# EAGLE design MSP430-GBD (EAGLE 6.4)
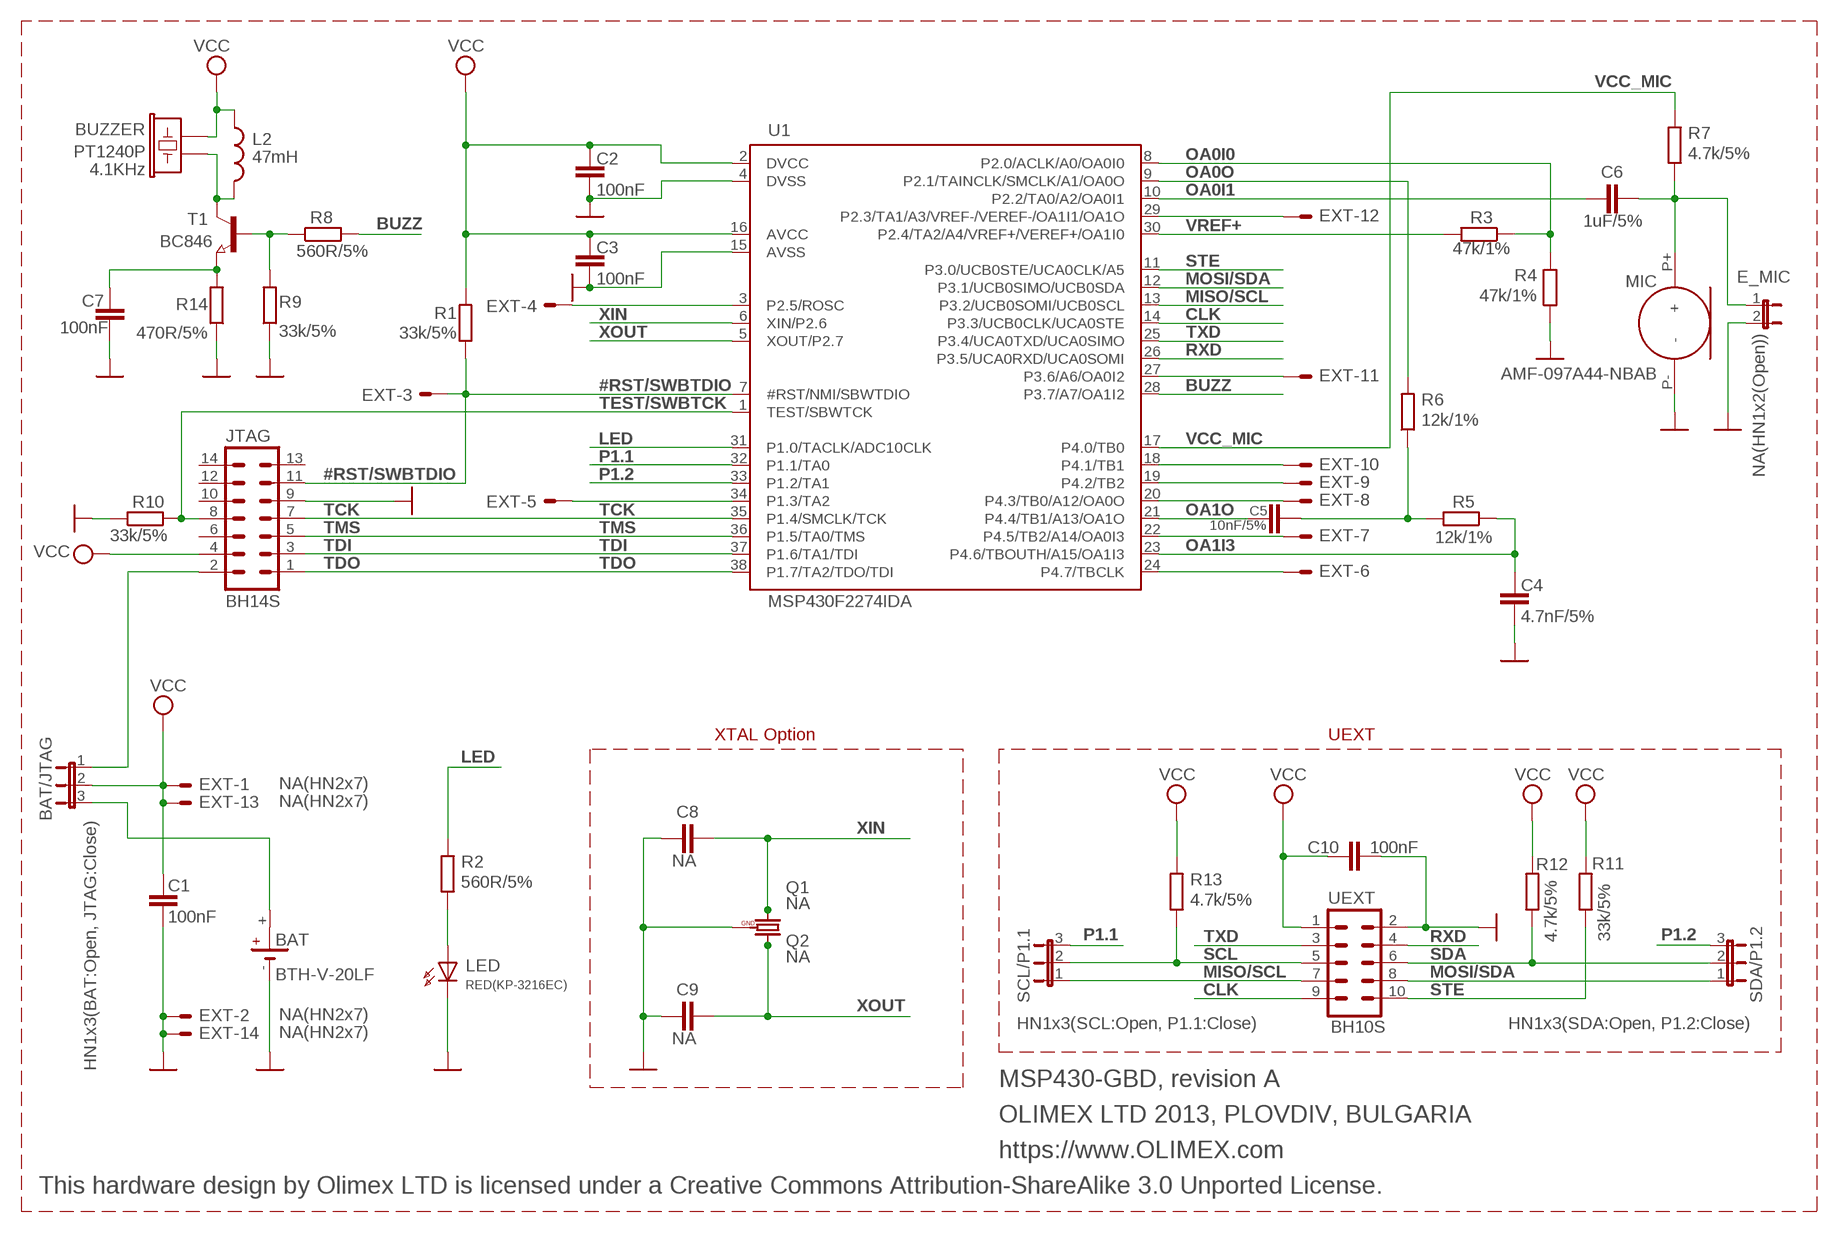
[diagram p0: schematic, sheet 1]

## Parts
BAT  BTH-V-20LF  B1  [3V_BAT_HOLDER]
BAT/JTAG  HN1x3(BAT:Open, JTAG:Close)  JP2E  [JP2]
BUZZER  PT1240P  BUZ3  [BUZ14MM]
C1  100nF  C-EUC0603  [C0603]
C2  100nF  C-EUC0603  [C0603]
C3  100nF  C-EUC0603  [C0603]
C4  4.7nF/5%  C-EUC0603  [C0603]
C5  10nF/5%  C-EUC0603  [C0603]
C6  1uF/5%  C-EUC0603  [C0603]
C7  100nF  C-EUC0603  [C0603]
C8  NA  C-EUC0603  [C0603]
C9  NA  C-EUC0603  [C0603]
C10  100nF  C-EUC0603  [C0603]
E_MIC  NA(HN1x2(Open))  JP1E  [JP1]
EXT  NA(HN2x7)  ML14ML14_NO_FRAMEE  [ML14_NO_FRAME]
JTAG  BH14S  ML14  [ML14]
L2  47mH  LSW68  [SW68]
LED  RED(KP-3216EC)  LED2  [SMD_LED]
MIC  AMF-097A44-NBAB  MICR  [MIC]
Q1  NA  HC49/S2  [HC49/SMD2]
Q2  NA  Q_GNDTC38H_SMD_GND  [TC38H_SMD_GND]
R1  33k/5%  R-EU_R0603  [R0603]
R2  560R/5%  R-EU_R0603  [R0603]
R3  47k/1%  R-EU_R0603  [R0603]
R4  47k/1%  R-EU_R0603  [R0603]
R5  12k/1%  R-EU_R0603  [R0603]
R6  12k/1%  R-EU_R0603  [R0603]
R7  4.7k/5%  R-EU_R0603  [R0603]
R8  560R/5%  R-EU_R0603  [R0603]
R9  33k/5%  R-EU_R0603  [R0603]
R10  33k/5%  R-EU_R0603  [R0603]
R11  33k/5%  R-EU_R0603  [R0603]
R12  4.7k/5%  R-EU_R0603  [R0603]
R13  4.7k/5%  R-EU_R0603  [R0603]
R14  470R/5%  R-EU_R1206_5MIL_WS  [R1206_5MIL_WS]
SCL/P1.1  HN1x3(SCL:Open, P1.1:Close)  JP2E  [JP2]
SDA/P1.2  HN1x3(SDA:Open, P1.2:Close)  JP2E  [JP2]
T1  BC846  NPN-TRANSISTOR_SOT23  [SOT23]
U1  MSP430F2274IDA  MSP430F2274  [TSSOP38]
UEXT  BH10S  ML10  [ML10]

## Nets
#RST/SWBTDIO: EXT.3 JTAG.11 R1.1 U1.7(#RST/NMI/SBWTDIO)
BUZZ: R8.2 U1.28(P3.7/A7/OA1I2)
CLK: U1.14(P3.3/UCB0CLK/UCA0STE) UEXT.9
GND: BAT.- C1.2 C2.2 C3.2 C4.2 C7.1 C8.1 C9.1 C10.2 E_MIC.2 EXT.2 EXT.14 JTAG.9 LED.C MIC.P-(-) Q2.GND R4.1 R9.1 R10.1 R14.1 U1.4(DVSS) U1.15(AVSS) UEXT.2
LED: R2.2 U1.31(P1.0/TACLK/ADC10CLK)
MISO/SCL: SCL/P1.1.1 U1.13(P3.2/UCB0SOMI/UCB0SCL) UEXT.7
MOSI/SDA: SDA/P1.2.1 U1.12(P3.1/UCB0SIMO/UCB0SDA) UEXT.8
N$1: BAT.+ BAT/JTAG.3
N$2: BAT/JTAG.1 JTAG.2
N$3: EXT.4 U1.3(P2.5/ROSC)
N$4: LED.A R2.1
N$6: C6.2 E_MIC.1 MIC.P+(+) R7.1
N$7: C5.2 R5.2 R6.1
N$9: R8.1 R9.2 T1.1(B)
N$10: C7.2 R14.2 T1.2(E)
N$14: EXT.5 U1.34(P1.3/TA2)
N$19: EXT.6 U1.24(P4.7/TBCLK)
N$20: BUZZER.+ L2.2 T1.3(C)
N$21: EXT.7 U1.22(P4.5/TB2/A14/OA0I3)
N$22: EXT.8 U1.20(P4.3/TB0/A12/OA0O)
N$23: EXT.9 U1.19(P4.2/TB2)
N$24: EXT.10 U1.18(P4.1/TB1)
N$25: EXT.11 U1.27(P3.6/A6/OA0I2)
N$26: EXT.12 U1.29(P2.3/TA1/A3/VREF-/VEREF-/OA1I1/OA1O)
OA0I0: R3.1 R4.2 U1.8(P2.0/ACLK/A0/OA0I0)
OA0I1: C6.1 U1.10(P2.2/TA0/A2/OA0I1)
OA0O: R6.2 U1.9(P2.1/TAINCLK/SMCLK/A1/OA0O)
OA1I3: C4.1 R5.1 U1.23(P4.6/TBOUTH/A15/OA1I3)
OA1O: C5.1 U1.21(P4.4/TB1/A13/OA1O)
P1.1: SCL/P1.1.3 U1.32(P1.1/TA0)
P1.2: SDA/P1.2.3 U1.33(P1.2/TA1)
RXD: U1.26(P3.5/UCA0RXD/UCA0SOMI) UEXT.4
SCL: R13.1 SCL/P1.1.2 UEXT.5
SDA: R12.1 SDA/P1.2.2 UEXT.6
STE: R11.1 U1.11(P3.0/UCB0STE/UCA0CLK/A5) UEXT.10
TCK: JTAG.7 U1.35(P1.4/SMCLK/TCK)
TDI: JTAG.3 U1.37(P1.6/TA1/TDI)
TDO: JTAG.1 U1.38(P1.7/TA2/TDO/TDI)
TEST/SWBTCK: JTAG.8 R10.2 U1.1(TEST/SBWTCK)
TMS: JTAG.5 U1.36(P1.5/TA0/TMS)
TXD: U1.25(P3.4/UCA0TXD/UCA0SIMO) UEXT.3
VCC: BAT/JTAG.2 BUZZER.- C1.1 C2.1 C3.1 C10.1 EXT.1 EXT.13 JTAG.4 L2.1 R1.2 R11.2 R12.2 R13.2 U1.2(DVCC) U1.16(AVCC) UEXT.1
VCC_MIC: R7.2 U1.17(P4.0/TB0)
VREF+: R3.2 U1.30(P2.4/TA2/A4/VREF+/VEREF+/OA1I0)
XIN: C8.2 Q1.2 Q2.1 U1.6(XIN/P2.6)
XOUT: C9.2 Q1.1 Q2.2 U1.5(XOUT/P2.7)
Unconnected: BAT.1+(+) JTAG.6 JTAG.10 JTAG.12 JTAG.13 JTAG.14

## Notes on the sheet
- PT1240P
- 4.1KHz
- XTAL Option | UEXT
- MSP430-GBD, revision A
- OLIMEX LTD 2013, PLOVDIV, BULGARIA
- https://www.OLIMEX.com
- This hardware design by Olimex LTD is licensed under a Creative Commons Attribution-ShareAlike 3.0 Unported License.

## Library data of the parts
BAT = DOUBLE-SIDE:B: LI BATTERY Varta
BAT/JTAG SCL/P1.1 SDA/P1.2 = jumper:JP2E: JUMPER
BUZZER = gogo:BUZ
C1-C10 = rcl:C-EU: CAPACITOR, European symbol
E_MIC = jumper:JP1E: JUMPER
EXT = con-harting-ml:ML14?E: HARTING
JTAG = con-harting-ml:ML14: HARTING
L2 = DOUBLE-SIDE:L
LED = DOUBLE-SIDE:LED
MIC = DOUBLE-SIDE:MIC: ELECTRETE MICROPHONE
Q1 = crystal:HC49/S: CRYSTAL
Q2 = crystal:Q_GND
R1-R14 = rcl:R-EU_: RESISTOR, European symbol
T1 = semicon-smd-ipc:NPN-TRANSISTOR_: NPN TRANSISTOR
U1 = OLIMEX_IC:MSP430F2274
UEXT = con-harting-ml:ML10: HARTING

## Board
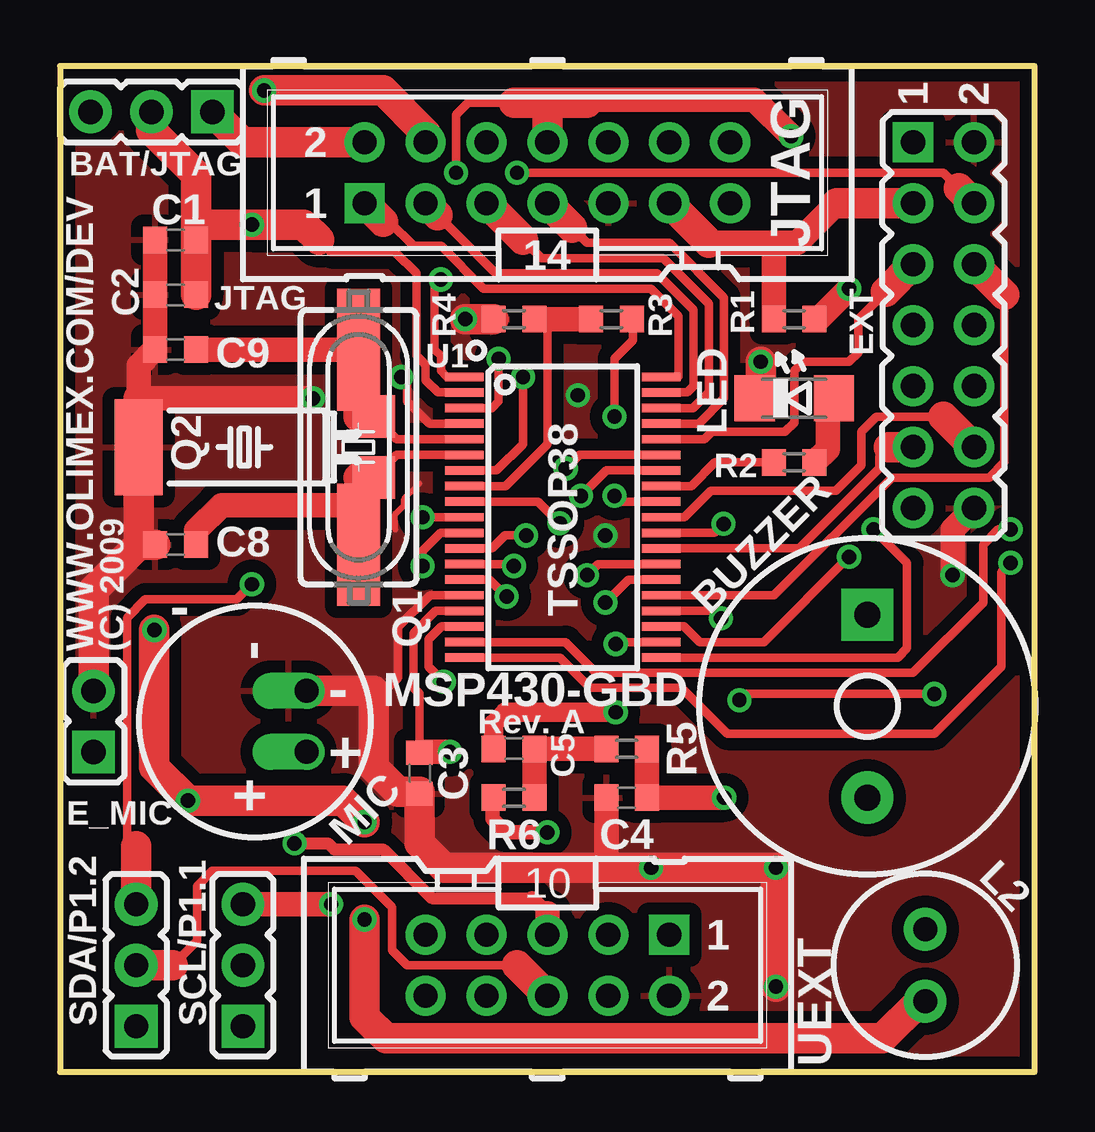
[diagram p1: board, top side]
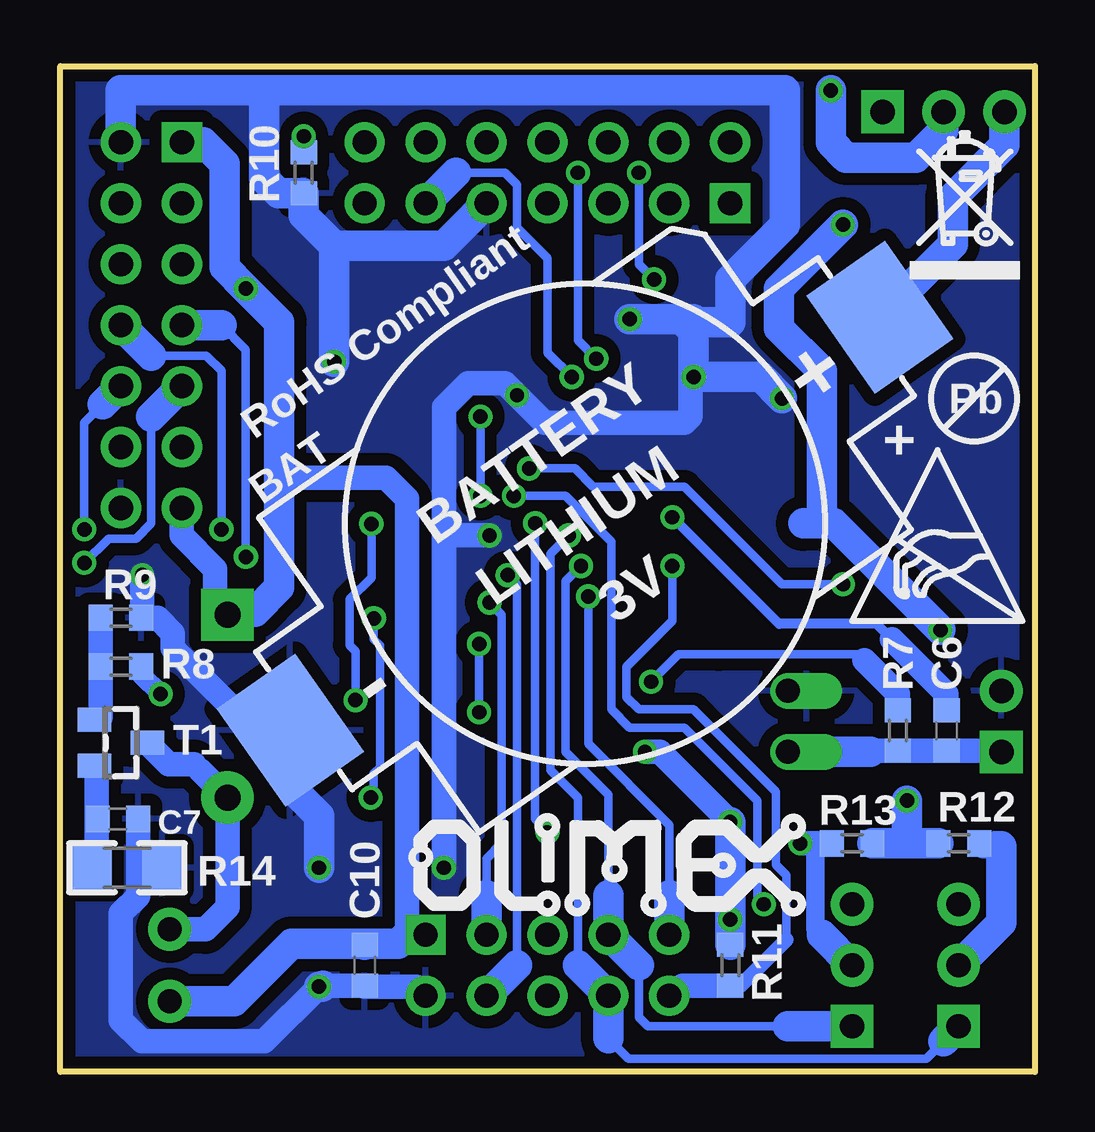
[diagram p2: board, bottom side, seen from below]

Size 40.62 x 41.91 mm. Coordinates in mm from the lower left corner, seen from the top.
Outline: 0.01,0 40.62,0 40.62,41.91 0.01,41.91 0,41.91 0,0.01 0.01,0
Copper layers (1+16): Top 0.035mm / dielectric 1.5mm / Bottom 0.035mm
Design rules "default": minimum track width 10mil, minimum drill 23mil, track to track 10mil, track to pad 10mil, pad to pad 10mil, via to via 10mil, smd to smd 0mil, copper to edge 10mil, drill to drill 10mil, minimum pad ring 10mil, minimum via ring 8mil, stop-mask expansion 4mil, vias tented up to drill 25mil, thermal gap 20mil

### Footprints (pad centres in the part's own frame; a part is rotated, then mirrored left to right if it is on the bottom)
3V_BAT_HOLDER = smd 2 x 2: 1+ -15,0 | smd 4 x 5: + -15,0; - 15,0
JP2 = drill 1.016 pad 1.778 square: 1 -2.54,0 | drill 1.016 pad 1.778: 2 0,0; 3 2.54,0
BUZ14MM = drill 1.092 pad 2.184: + 3.81,0 | drill 1.092 pad 2.184 square: - -3.81,0
C0603 = smd 1 x 1.1: 1 -0.85,0; 2 0.85,0
JP1 = drill 1.016 pad 1.778 square: 1 0,-1.27 | drill 1.016 pad 1.778: 2 0,1.27
ML14_NO_FRAME = drill 1.016 pad 1.676 square: 1 -7.62,-1.27 | drill 1.016 pad 1.676: 2 -7.62,1.27; 3 -5.08,-1.27; 4 -5.08,1.27; 5 -2.54,-1.27; 6 -2.54,1.27; 7 0,-1.27; 8 0,1.27; 9 2.54,-1.27; 10 2.54,1.27; 11 5.08,-1.27; 12 5.08,1.27; 13 7.62,-1.27; 14 7.62,1.27
ML14 = drill 1.016 pad 1.676 square: 1 -7.62,-1.27 | drill 1.016 pad 1.676: 2 -7.62,1.27; 3 -5.08,-1.27; 4 -5.08,1.27; 5 -2.54,-1.27; 6 -2.54,1.27; 7 0,-1.27; 8 0,1.27; 9 2.54,-1.27; 10 2.54,1.27; 11 5.08,-1.27; 12 5.08,1.27; 13 7.62,-1.27; 14 7.62,1.27
SW68 = drill 1 pad 1.778: 1 -1.5,0; 2 1.5,0
SMD_LED = smd 1.676 x 1.93: A 1.65,0; C -1.65,0
MIC = drill 1 offset: P+ -1.27,-2.159; P- 1.27,-2.159
HC49/SMD2 = smd 5.08 x 1.778: 1 -4.064,0; 2 4.064,0
TC38H_SMD_GND = smd 1.778 x 1.778: 1 -1.27,-3.81; 2 1.27,-3.81 | smd 4 x 2: GND 0,6
R0603 = smd 1 x 1.1: 1 -0.85,0; 2 0.85,0
R1206_5MIL_WS = smd 1.651 x 1.778: 1 -1.46,0; 2 1.46,0
SOT23 = smd 1 x 1.4: 1 -0.95,-1.1; 2 0.95,-1.1; 3 0,1.1
TSSOP38 = smd 0.35 x 1.6: 1 -5.85,-4.1; 2 -5.2,-4.1; 3 -4.55,-4.1; 4 -3.9,-4.1; 5 -3.25,-4.1; 6 -2.6,-4.1; 7 -1.95,-4.1; 8 -1.3,-4.1; 9 -0.65,-4.1; 10 0,-4.1; 11 0.65,-4.1; 12 1.3,-4.1; 13 1.95,-4.1; 14 2.6,-4.1; 15 3.25,-4.1; 16 3.9,-4.1; 17 4.55,-4.1; 18 5.2,-4.1; 19 5.85,-4.1; 20 5.85,4.1; 21 5.2,4.1; 22 4.55,4.1; 23 3.9,4.1; 24 3.25,4.1; 25 2.6,4.1; 26 1.95,4.1; 27 1.3,4.1; 28 0.65,4.1; 29 0,4.1; 30 -0.65,4.1; 31 -1.3,4.1; 32 -1.95,4.1; 33 -2.6,4.1; 34 -3.25,4.1; 35 -3.9,4.1; 36 -4.55,4.1; 37 -5.2,4.1; 38 -5.85,4.1
ML10 = drill 1.016 pad 1.676 square: 1 -5.08,-1.27 | drill 1.016 pad 1.676: 2 -5.08,1.27; 3 -2.54,-1.27; 4 -2.54,1.27; 5 0,-1.27; 6 0,1.27; 7 2.54,-1.27; 8 2.54,1.27; 9 5.08,-1.27; 10 5.08,1.27

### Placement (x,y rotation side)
BAT  18.75,22.84 215 bottom
BAT/JTAG  3.81,40.01 180 top
BUZZER  33.66,15.24 270 top
C1  4.83,34.67 180 top
C2  4.83,32.38 180 top
C3  14.99,12.45 270 top
C4  23.62,11.43 180 top
C5  18.92,13.46 0 top
C6  3.68,14.22 270 bottom
C7  38.23,10.54 180 bottom
C8  4.83,21.97 0 top
C9  4.83,30.1 0 top
C10  27.94,4.45 270 bottom
E_MIC  1.4,14.61 0 top
EXT  36.83,31.11 270 top
JTAG  20.32,37.47 0 top
L2  36.07,4.45 90 top
LED  30.61,28.07 0 top
MIC  8.13,14.61 90 top
Q1  12.45,26.04 270 top
Q2  9.27,26.04 90 top
R1  30.61,31.37 0 top
R2  30.61,25.4 180 top
R3  22.99,31.37 0 top
R4  18.92,31.37 0 top
R5  23.62,13.46 180 top
R6  18.92,11.43 180 top
R7  5.71,14.22 90 bottom
R8  38.1,16.89 0 bottom
R9  38.1,18.92 180 bottom
R10  30.48,37.47 90 bottom
R11  12.7,4.45 90 bottom
R12  3.17,9.53 180 bottom
R13  7.62,9.53 0 bottom
R14  37.85,8.51 180 bottom
SCL/P1.1  7.62,4.45 90 top
SDA/P1.2  3.17,4.45 90 top
T1  38.1,13.72 270 bottom
U1  20.95,23.11 270 top
U$1  [RECYCLE_BIN1/8]  5.21,33.02 0 bottom
U$3  [PB_SMALL]  2.54,28.07 0 bottom
U$4  [ESD_SYMBOL]  7.62,18.8 0 bottom
U$6  [OLIMEX_LOGO1_V]  8.38,6.35 0 bottom
UEXT  20.32,4.45 180 top

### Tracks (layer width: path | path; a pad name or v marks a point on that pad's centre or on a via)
#RST/SWBTDIO  (via drill 0.6)
  Top 0.356: U1.7 18.21,25.06 19.3,26.16 v19.3,28.96
  Top 1.016: 27.05,34.54 29.76,34.54 | 29.76,34.54 30.73,34.54 32.38,36.2 | 29.76,34.54 R1.1
  Top 1.27: JTAG.11 27.05,34.54 | 32.38,36.2 EXT.3
  Bottom 0.356: 24.13,37.47 22.1,37.47 21.59,36.96 21.59,35.18 20.32,33.91 20.32,29.97 v19.3,28.96
  Bottom 1.27: 24.13,37.47 JTAG.11
BUZZ  (via drill 0.6)
  Top 0.356: U1.28 27.29,22.46 v27.66,22.84 | v28.32,15.49 28.57,15.75 v36.45,15.75
  Bottom 0.356: v28.32,15.49 28.32,17.53 28.57,17.78 28.57,19.68 27.66,20.6 v27.66,22.84
  Bottom 0.813: v36.45,15.75 37.25,16.55 R8.2
CLK  (via drill 0.6)
  Top 0.356: U1.14 17.92,20.51 v18.62,19.81
  Bottom 0.356: v18.62,19.81 18.62,13.66 15.24,10.29 15.24,7.37
  Bottom 1.27: UEXT.9 15.24,7.37
GND  (via drill 0.6)
  Top 0.254: 14.99,24.51 14.35,23.88 14.35,23.62 13.97,23.24 13.97,22.61
  Top 0.356: U1.4 15.4,27.01 14.48,27.94 14.48,28.7 v14.22,28.96 | U1.15 15.42,19.86 14.1,18.54 14.1,16.43 13.54,15.88 13.08,15.88
  Top 1.016: C1.2 C2.2 C9.1 3.94,30.1 3.27,29.43 3.27,28.07 v10.54,28.07 | 29.21,28.07 LED.C | 22.73,8.51 22.77,8.51 C4.2 | EXT.14 37.21,22.61 v37.21,20.7
  Top 1.27: 3.27,28.07 Q2.GND 3.27,21.97 | 3.27,21.97 C8.1 | 3.27,21.97 1.4,20.1 E_MIC.2 | v29.21,29.59 29.21,28.07 | v29.84,3.56 v29.84,8.51 v24.64,8.51 22.73,8.51 16,8.51 14.99,9.53 C3.2 14.99,11.68 14.1,11.68 13.08,12.7 13.08,15.88 MIC.P- | v16.89,31.37 R4.1
  Bottom 0.356: 38.1,2.16 38.1,2.29
  Bottom 0.813: 28.16,3.6 28.07,3.68 27.98,3.6 C10.2 27.94,3.56 | 23.5,28.7 23.62,28.7
  Bottom 1.016: 37.21,18.92 36.58,18.92 35.94,18.29 35.94,17.65 32.53,14.24 BAT.- | v14.22,28.96 14.35,28.96 14.35,27.3 14.61,27.05 20.45,27.05 v21.59,28.19 22.1,28.7 23.5,28.7 | 24.64,22.35 v22.73,22.35 | 24.64,22.35 v24.64,8.51 | v29.84,3.56 32.13,1.27 37.21,1.27 38.1,2.16 | 38.1,2.29 38.1,6.6 37.38,7.33 37.38,8.51 | 37.38,8.51 C7.1 | 37.21,18.92 R9.1 | 37.21,18.92 v37.21,20.7 | 29.68,3.6 28.16,3.6 | UEXT.2 25.78,3.56 27.94,3.56 | 37.38,8.51 R14.1 | 24.64,22.35 24.64,27.69 23.62,28.7
  Bottom 1.27: v10.54,28.07 11.43,28.96 v14.22,28.96 14.22,31.37 14.48,31.37 | 32.13,40.89 10.41,40.89 10.41,35.31 12.7,33.02 12.7,31.24 14.35,31.24 14.48,31.11 14.48,31.37 | 32.13,40.89 38.1,40.89 EXT.2 | 32.13,40.89 32.13,37.21 31.54,36.62 R10.1 30.48,35.69 29.21,34.42 | JTAG.9 24.64,34.42 29.21,34.42 | 14.48,31.37 v16.89,31.37 | 29.21,34.42 v29.21,29.59 | v29.84,8.51 29.84,10.67 30.99,11.81 30.99,14.22 31.02,14.22 BAT.- | v29.84,3.56 29.72,3.56 29.68,3.6
  pour Top (isolate 0.508, rank 3): -2.54,43.18 42.93,43.18 42.93,-2.54 -2.54,-2.54
  pour Bottom (isolate 0.508, rank 3): -2.54,45.72 43.81,45.72 43.81,-2.54 -2.54,-2.54
LED
  Top 0.356: U1.31 26.32,24.41 27.3,25.4 R2.2
MISO/SCL  (via drill 0.6)
  Top 0.356: U1.13 18.85,21.16 18.93,21.08 v18.92,21.08
  Bottom 0.356: v18.92,21.08 19.56,20.45 19.56,13.34 17.78,11.56 17.78,7.37 | 16.51,4.45 16.51,2.29 16.13,1.91 10.29,1.91
  Bottom 1.27: 17.78,7.37 UEXT.7 16.51,4.45 | SCL/P1.1.1 10.29,1.91
MOSI/SDA  (via drill 0.6)
  Top 0.356: U1.12 18,21.81 18.54,22.35 v19.43,22.35
  Bottom 0.356: v19.43,22.35 20.19,21.59 20.19,12.57 19.05,11.43 19.05,4.45 | 3.81,1.27 4.52,0.56 16.94,0.56 17.78,1.4
  Bottom 1.27: 19.05,4.45 UEXT.8 17.78,1.4 | SDA/P1.2.1 3.81,1.27
N$1
  Bottom 1.27: BAT/JTAG.3 1.27,38.61 3.43,36.45 3.43,34.48 BAT.+
N$2
  Top 1.27: BAT/JTAG.1 7.62,38.73 JTAG.2
N$3  (via drill 0.6)
  Top 0.356: U1.3 18.01,27.66 18.29,27.94 v18.29,29.72 | v19.05,37.47 36.83,37.47 37.47,36.83
  Top 1.27: 37.47,36.83 EXT.4
  Bottom 0.356: v18.29,29.72 19.05,30.48 v19.05,37.47
N$4
  Top 1.016: R2.1 32,25.95 32,27.81 LED.A
N$6
  Bottom 1.016: 6.86,13.34 6.82,13.37 R7.1 C6.2 1.82,13.37 1.78,13.34 E_MIC.1
  Bottom 1.27: 6.86,13.34 MIC.P+
N$7
  Top 1.016: R5.2 C5.2 R6.1
N$9
  Bottom 1.016: R9.2 R8.1 38.95,14.77 39.05,14.67 T1.1
N$10
  Bottom 1.016: T1.2 39.12,12.77 39.12,10.29 | R14.2 39.31,8.95 39.12,9.14 39.12,10.29 | 39.12,10.29 39.12,10.54 C7.2 39.08,10.33 39.12,10.29
N$14
  Top 0.356: U1.34 26.87,26.36 27.18,26.67 30.23,26.67 30.61,27.05 30.61,29.21 30.99,29.59 32.89,29.59 33.27,29.97 33.27,31.37 34.42,32.51
  Top 1.27: 34.42,32.51 EXT.5
N$19
  Top 0.356: 39.37,32.38 39.37,25.4 38.73,24.77 34.67,24.77 29.77,19.86 U1.24
  Top 1.27: 39.37,32.38 EXT.6
N$20
  Bottom 0.762: 34.8,12.57 35.05,12.83
  Bottom 1.016: 34.8,12.57 BUZZER.+ 33.66,6.86 34.57,5.95 L2.2 | 35.05,12.83 36.11,12.83 T1.3
N$21  (via drill 0.6)
  Top 0.356: U1.22 26.01,18.56 26.67,17.91 29.34,17.91 v32.89,21.46
  Bottom 0.356: v32.89,21.46 32.89,30.1 33.91,31.11
  Bottom 1.27: 33.91,31.11 EXT.7
N$22  (via drill 0.6)
  Top 0.356: U1.20 34.92,17.26 35.31,17.65 35.31,21.21 v33.91,22.61
  Bottom 0.356: v33.91,22.61 33.91,29.21 34.54,29.84 36.83,29.84
  Bottom 1.27: 36.83,29.84 EXT.8
N$23  (via drill 0.6)
  Top 0.356: U1.19 20.84,17.26 22.1,16 25.91,16 27.81,14.1 36.45,14.1 39.24,16.89 39.24,20.83 v39.62,21.21
  Bottom 0.356: v39.62,21.21 38.61,22.23 37.47,22.23 36.83,22.86 36.83,27.3
  Bottom 1.27: 36.83,27.3 EXT.9
N$24  (via drill 0.6)
  Top 0.356: U1.18 21.07,17.91 22.35,16.64 35.56,16.64 38.48,19.56 38.48,21.97 39.12,22.61 v39.62,22.61
  Bottom 0.356: v39.62,22.61 39.62,27.05 38.86,27.81
  Bottom 1.27: 38.86,27.81 EXT.10
N$25
  Top 0.356: U1.27 30.83,21.81 34.16,25.15 34.16,25.65 34.54,26.04
  Top 1.27: 34.54,26.04 EXT.11
N$26
  Top 0.356: U1.29 26.04,23.11 27.13,24.21 32.33,24.21 33.4,25.27 33.4,26.67 34.04,27.3 36.83,27.3
  Top 1.27: 36.83,27.3 EXT.12
OA0I0
  Top 0.356: U1.8 18.57,24.41 20.32,26.16 20.32,31.37 R4.2
  Top 1.016: R4.2 R3.1
OA0I1  (via drill 0.6)
  Top 0.356: v15.11,23.11 U1.10
  Bottom 0.406: 5.97,18.03 6.6,18.67 10.67,18.67 v15.11,23.11
  Bottom 1.016: C6.1 3.68,15.75 5.97,18.03
OA0O  (via drill 0.6)
  Top 0.356: U1.9 19.92,23.76 v20.83,22.86
  Top 0.61: R6.2 18.07,11.34 18.03,11.3 18.03,10.54 18.59,9.98 v20.32,9.98
  Bottom 0.356: v20.83,22.86 20.83,10.54 20.32,10.03 v20.32,9.98
OA1I3  (via drill 0.6)
  Top 0.356: U1.23 27.24,19.21 v27.56,18.9
  Top 1.016: v27.69,11.43 C4.1 24.47,12.45 R5.1
  Bottom 0.356: v27.56,18.9 27.56,18.03 27.3,17.78 27.3,12.7 27.56,12.45 27.56,11.43 v27.69,11.43
OA1O  (via drill 0.6)
  Top 0.356: U1.21 23.25,17.91 v23.16,17.83
  Top 0.61: v23.16,14.99 23.16,15.06 23.11,15.11 22.99,14.99
  Top 0.813: C5.1 18.07,14.52 18.54,14.99 22.99,14.99
  Bottom 0.356: v23.16,14.99 v23.16,17.83
P1.1  (via drill 0.6)
  Top 0.356: U1.32 22.78,25.06 v21.72,24
  Top 1.016: SCL/P1.1.3 v11.3,6.99
  Bottom 0.356: v11.3,6.99 11.56,7.24 11.56,11.3 14.61,14.35 16.89,14.35 17.65,15.11 17.65,22.1 19.56,24 v21.72,24
P1.2  (via drill 0.6)
  Top 0.356: U1.33 21.65,25.71 v21.08,25.15 | v8,20.32 7.37,19.68 3.56,19.68 2.79,18.92 2.79,9.78 3.17,9.4
  Top 1.27: SDA/P1.2.3 3.17,9.4
  Bottom 0.356: v8,20.32 10.54,20.32 14.61,24.38 18.41,24.38 19.18,25.15 v21.08,25.15
RXD  (via drill 0.6)
  Top 0.356: U1.26 22.43,21.16 v21.97,20.7
  Bottom 0.356: 21.59,4.45 21.59,20.32 v21.97,20.7
  Bottom 1.27: 21.59,4.45 UEXT.4
SCL  (via drill 0.6)
  Top 0.508: 19.68,7.24 15.49,7.24 13.46,9.27 11.43,9.27 11.18,9.53 v9.78,9.53
  Top 0.61: 19.68,7.24 20.32,6.6
  Top 1.016: 20.32,6.6 UEXT.5
  Bottom 0.762: 8.89,5.71 9.14,5.97 9.14,9.53
  Bottom 1.016: v9.78,9.53 9.14,9.53 R13.1
  Bottom 1.27: SCL/P1.1.2 8.89,5.71
SDA
  Top 0.356: 19.05,4.45 14.48,4.45 13.84,5.08 13.84,6.86 12.32,8.38 6.35,8.38 5.71,7.75 5.71,5.46 4.7,4.45
  Top 1.27: 19.05,4.45 UEXT.6 | SDA/P1.2.2 4.7,4.45
  Bottom 1.016: R12.1 2.29,9.53 2.16,9.4 1.65,9.4
  Bottom 1.27: SDA/P1.2.2 1.4,6.22 1.4,9.4 1.65,9.4
STE  (via drill 0.6)
  Top 0.356: U1.11 15.86,22.46 15.11,21.72 v15.11,21.08
  Bottom 0.356: 12.45,3.56 12.32,3.56 12.28,3.6 R11.1 | v15.11,21.08 15.11,18.8 17.02,16.89 17.02,15.62 16.51,15.11 14.22,15.11 10.79,11.68 10.79,8.64 10.36,8.2 10.36,5.51
  Bottom 0.61: 12.28,3.6 10.36,5.51
  Bottom 1.016: UEXT.10 15.11,3.17 14.69,3.6 R11.1
TCK
  Top 0.356: U1.35 26.63,27.01 27.69,28.07 27.69,32.26 25.4,34.54 21.97,34.54 21.34,35.18
  Top 1.27: 21.34,35.18 JTAG.7
TDI
  Top 0.356: U1.37 26.16,28.31 26.42,28.57 26.42,31.75 24.89,33.27 18.16,33.27 15.75,35.69
  Top 1.27: JTAG.3 15.75,35.69
TDO
  Top 0.356: U1.38 25.78,28.96 25.78,31.5 24.64,32.64 17.65,32.64 15.88,34.42 14.73,34.42 13.72,35.43 13.46,35.43
  Top 1.27: 13.46,35.43 JTAG.1
TEST/SWBTCK  (via drill 0.6)
  Top 0.356: U1.1 16.12,28.96 15.88,29.21 15.88,29.84 15.62,30.1 15.62,32.77 v15.88,33.02 | v16.51,37.47 16.51,39.88 17.02,40.39 18.92,40.39
  Top 1.016: 21.97,40.39 22.1,40.51 28.96,40.51 v30.48,38.99
  Top 1.27: 18.92,40.39 20.32,40.39 | 20.32,40.39 JTAG.8 | 20.32,40.39 21.97,40.39
  Bottom 0.356: v16.51,37.47 16.51,33.66 v15.88,33.02
  Bottom 1.016: v30.48,38.99 R10.2
TMS
  Top 0.356: U1.36 26.39,27.66 27.05,28.32 27.05,32 25.15,33.91 20.07,33.91 19.3,34.67
  Top 1.27: 19.3,34.67 JTAG.5
TXD  (via drill 0.6)
  Top 0.356: U1.25 23.69,20.51 v22.73,19.56
  Bottom 0.356: v22.73,19.56 22.23,19.05 22.23,9.53 22.86,8.89 22.86,7.37
  Bottom 1.27: UEXT.3 22.86,7.37
VCC  (via drill 0.6)
  Top 0.356: 10.79,34.67 11.3,34.16 13.97,34.16 14.86,33.27 14.86,29.84 15.24,29.46 15.24,28.83 15.76,28.31 U1.2 | U1.16 15.66,19.21 14.73,18.29 14.73,16 14.99,15.75 14.99,13.34
  Top 1.016: v32.89,32.64 31.62,31.37 R1.2 | v16.26,13.34 14.99,13.34 C3.1
  Top 1.27: 10.79,34.67 10.16,35.31 v8,35.31 5.68,35.31 | C2.1 C1.1 5.68,35.31 | BAT/JTAG.2 3.81,39.24 5.68,37.38 5.68,35.31 | v12.7,10.41 11.81,11.3 v5.33,11.3 3.94,12.7 v3.94,18.41 | v12.7,6.35 12.7,2.29 13.59,1.4 34.29,1.4 35.84,2.94 L2.1 | JTAG.4 15.24,39.12 13.46,40.89 v8.51,40.89
  Bottom 1.016: EXT.13 35.56,22.35 34.16,20.95 34.16,19.05 BUZZER.- | v12.7,10.41 15.62,13.34 v16.26,13.34 | 26.16,5.71 26.16,23.88 27.05,24.77 31.5,24.77
  Bottom 1.27: EXT.1 34.67,38.73 33.78,37.85 33.78,33.53 v32.89,32.64 31.5,31.24 31.5,24.77 31.5,20.19 32.51,19.18 33.66,19.18 BUZZER.- | R12.2 5.33,9.53 | 5.33,9.53 v5.33,11.3 | 5.33,9.53 R13.2 | v12.7,10.41 v12.7,6.35 R11.2 | 8.89,22.86 9.65,22.86 | v8.51,40.89 8.51,38.73 7.87,38.1 4.95,38.1 3.81,39.24 BAT/JTAG.2 | v8,35.31 10.67,32.64 10.67,30.99 8.89,29.21 8.89,22.86 | v3.94,18.41 8.38,22.86 8.89,22.86 | 28.07,5.33 30.99,5.33 33.38,2.94 L2.1 | UEXT.1 26.16,5.71 26.54,5.33 28.07,5.33 | 28.07,5.33 27.98,5.33 C10.1
VCC_MIC  (via drill 0.6)
  Top 0.356: U1.17 15.9,18.56 15.37,18.03 15.37,16.89 v16,16.26
  Bottom 0.356: 13.21,17.4 14.86,17.4 v16,16.26 | 13.21,17.4 13.16,17.4 | 7.11,17.14 7.37,17.4 13.21,17.4
  Bottom 1.016: 7.11,17.14 5.71,15.75 R7.2
VREF+  (via drill 0.6)
  Top 0.356: U1.30 23.35,23.76 v23.11,24 | R3.2 23.88,31.33 23.88,30.48 23.11,29.72 v23.11,27.3
  Bottom 0.356: v23.11,24 v23.11,27.3
XIN
  Top 0.356: U1.6 14.03,25.71 Q2.1
  Top 1.016: 12.45,24.77 12.45,23.62 6.73,23.62 5.68,22.57 C8.2
  Top 1.27: 12.45,24.77 Q2.1 | 12.45,23.62 Q1.2
XOUT
  Top 0.356: U1.5 14.02,26.36 Q2.2
  Top 1.016: C9.2 Q1.1
  Top 1.27: Q2.2 12.45,27.3 Q1.1

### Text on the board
tNames: - | WWW.OLIMEX.COM/DEV | (C) 2009 | - | MSP430-GBD | Rev. A | +
bNames: RoHS Compliant | +
bStop: WWW.OLIMEX.COM/DEV (C) 2009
